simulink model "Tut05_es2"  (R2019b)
settings: Solver=ode4  StartTime=0.0  StopTime=4  FixedStep=0.0001  RelTol=1e-3
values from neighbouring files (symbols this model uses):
  b = 0.1    [svolgimento.m]
  D = 0    [svolgimento.m]
  muC = 260    [svolgimento.m]
  Tc = 0.04    [svolgimento.m]

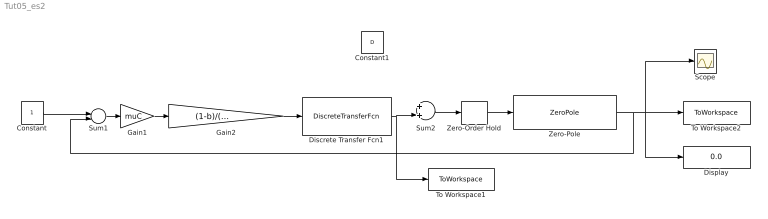
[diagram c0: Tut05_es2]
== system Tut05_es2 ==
  Constant : Constant
  Constant1 : Constant  Value=D
  Discrete Transfer Fcn1 : DiscreteTransferFcn  Numerator=[1 -0.9231]  Denominator=[1 -b]  SampleTime=Tc
  Display : Display
  Gain1 : Gain  Gain=muC
  Gain2 : Gain  Gain=(1-b)/(1-0.9231)
  Scope : Scope
  Sum1 : Sum  Inputs=+-
  Sum2 : Sum
  To Workspace1 : ToWorkspace  VariableName=u  SaveFormat=Timeseries  SampleTime=-1
  To Workspace2 : ToWorkspace  VariableName=y  SaveFormat=Timeseries  SampleTime=-1
  Zero-Order Hold : ZeroOrderHold  SampleTime=Tc
  Zero-Pole : ZeroPole  Zeros=[]  Poles=[-1 -2]  Gain=0.1
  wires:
  Zero-Pole/1 -> Scope/1, To Workspace2/1, Display/1, Sum1/2
  Sum1/1 -> Gain1/1
  Sum2/1 -> Zero-Order Hold/1
  Gain1/1 -> Gain2/1
  Zero-Order Hold/1 -> Zero-Pole/1
  Constant/1 -> Sum1/1
  Discrete Transfer Fcn1/1 -> To Workspace1/1, Sum2/2
  Gain2/1 -> Discrete Transfer Fcn1/1
